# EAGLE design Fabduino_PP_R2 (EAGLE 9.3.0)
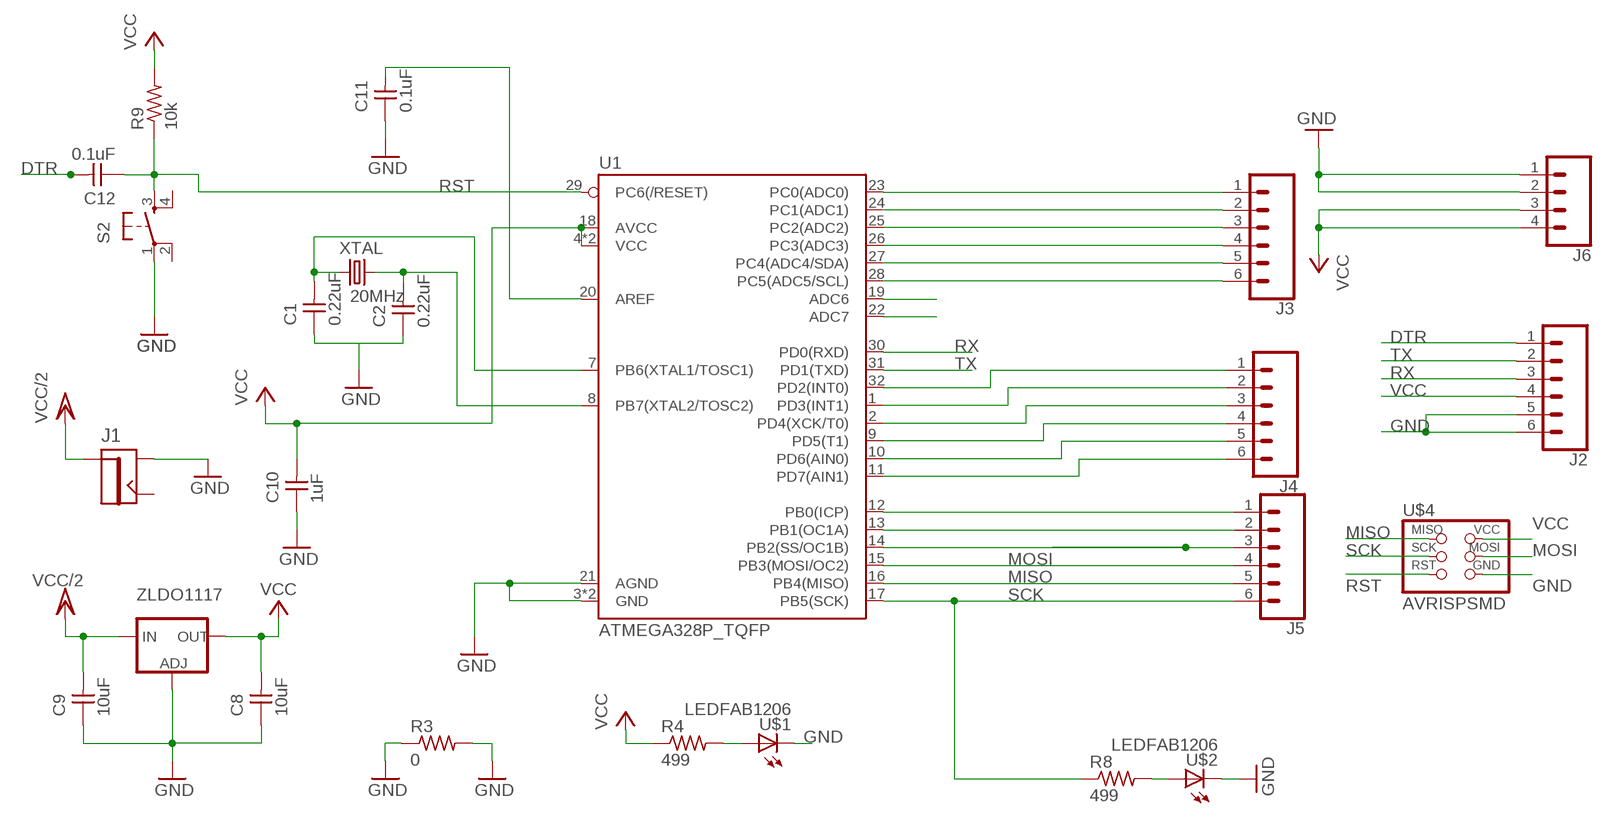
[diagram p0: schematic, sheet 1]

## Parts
C1  0.22uF  CAP-UNPOLARIZEDFAB  [C1206FAB]
C2  0.22uF  CAP-UNPOLARIZEDFAB  [C1206FAB]
C8  10uF  CAP-UNPOLARIZEDFAB  [C1206FAB]
C9  10uF  CAP-UNPOLARIZEDFAB  [C1206FAB]
C10  1uF  CAP-UNPOLARIZEDFAB  [C1206FAB]
C11  0.1uF  CAP-UNPOLARIZEDFAB  [C1206FAB]
C12  0.1uF  CAP-UNPOLARIZEDFAB  [C1206FAB]
J1  JACK.65MM  [JACK_.65MM]
J2  CONN_06SILK_FEMALE_PTH  [1X06]
J3  CONN_06SILK_FEMALE_PTH  [1X06]
J4  CONN_06SILK_FEMALE_PTH  [1X06]
J5  CONN_06SILK_FEMALE_PTH  [1X06]
J6  CONN_04PTH  [1X04]
R3  0  RES-US1206FAB  [R1206FAB]
R4  499  RES-US1206FAB  [R1206FAB]
R8  499  RES-US1206FAB  [R1206FAB]
R9  10k  RES-US1206FAB  [R1206FAB]
S2  6MM_SWITCH6MM_SWITCH  [6MM_SWITCH]
U1  ATMEGA328P_TQFP  [TQFP32-08]
U$1  LEDFAB1206  [LED1206FAB]
U$2  LEDFAB1206  [LED1206FAB]
U$4  AVRISPSMD  [2X03SMD]
XTAL  20MHz  CRYSTAL  [2-SMD-5X3MM]
ZLDO1117  V_REG_LM1117SOT223  [SOT223]

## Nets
DTR: C12.2 J2.1
GND: C1.1 C2.1 C8.1 C9.1 C10.1 C11.1 J1.CONTACT(SHUNT) J2.5 J2.6 J6.1 J6.2 R3.1 R3.2 S2.1(P) U1.3(GND) U1.5(GND) U1.21(AGND) U$1.2(C) U$2.2(C) U$4.6(GND) ZLDO1117.1(ADJ)
MISO: J5.5 U1.16(PB4(MISO)) U$4.1(MISO)
MOSI: J5.4 U1.15(PB3(MOSI/OC2)) U$4.4(MOSI)
N$2: J5.1 U1.12(PB0(ICP))
N$3: J3.1 U1.23(PC0(ADC0))
N$4: J3.2 U1.24(PC1(ADC1))
N$5: J3.3 U1.25(PC2(ADC2))
N$6: J3.4 U1.26(PC3(ADC3))
N$7: J3.5 U1.27(PC4(ADC4/SDA))
N$8: J3.6 U1.28(PC5(ADC5/SCL))
N$10: J4.1 U1.32(PD2(INT0))
N$11: J4.2 U1.1(PD3(INT1))
N$12: J4.3 U1.2(PD4(XCK/T0))
N$13: J4.4 U1.9(PD5(T1))
N$14: J4.5 U1.10(PD6(AIN0))
N$15: J4.6 U1.11(PD7(AIN1))
N$16: J5.2 U1.13(PB1(OC1A))
N$17: J5.3 U1.14(PB2(SS/OC1B))
N$18: C1.2 U1.7(PB6(XTAL1/TOSC1)) XTAL.P$1
N$19: C2.2 U1.8(PB7(XTAL2/TOSC2)) XTAL.P$2
N$20: C11.2 U1.20(AREF)
N$21: R4.2 U$1.1(A)
N$22: U1.19(ADC6)
N$23: R8.2 U$2.1(A)
N$24: U1.22(ADC7)
RST: C12.1 R9.1 S2.3(S) U1.29(PC6(/RESET)) U$4.5(RST)
RX: J2.3 U1.30(PD0(RXD))
SCK: J5.6 R8.1 U1.17(PB5(SCK)) U$4.3(SCK)
TX: J2.2 U1.31(PD1(TXD))
VCC: C8.2 C10.2 J2.4 J6.3 J6.4 R4.1 R9.2 U1.4(VCC) U1.6(VCC) U1.18(AVCC) U$4.2(VCC) ZLDO1117.2(OUT) ZLDO1117.4(OUT)
VCC/2: C9.2 J1.PIN ZLDO1117.3(IN)
Unconnected: J1.SHUNT(CONTACT) S2.2(P1) S2.4(S1)

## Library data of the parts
C1 C2 C8-C12 = fab:CAP-UNPOLARIZED
J1 = 01_fab:JACK
J2-J5 = SparkFun-Connectors:CONN_06: Multi connection point. Often used as Generic Header-pin footprint for 0.1 inch spaced/style header connections On any of the 0.1 inch spaced packages, you can populate with these: Break Away Headers - Straight (PRT-00116) Break Away Male Headers - Right Angle (PRT-00553) Female Headers (PRT-00115)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; PROD_ID: CONN-08437
J6 = SparkFun-Connectors:CONN_04: Multi connection point. Often used as Generic Header-pin footprint for 0.1 inch spaced/style header connections On any of the 0.1 inch spaced packages, you can populate with these: Break Away Headers - Straight (PRT-00116) Break Away Male Headers - Right Angle (PRT-00553) Female Headers (PRT-00115)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; PROD_ID: CONN-09696
R3 R4 R8 R9 = fab:RES-US: Resistor (US Symbol)
S2 = fab:6MM_SWITCH: OMRON SWITCH
U1 = SparkFun-IC-Microcontroller:ATMEGA328P_TQFP: Popular 328P in QFP Storefront component: ATmega328 - TQFP (COM-13448) Datasheet SparkFun Products SparkFun RedBoard - Programmed with Arduino (DEV-12757) Arduino Pro Mini 328 - 5V/16MHz (DEV-11113) Arduino Pro Mini 328 - 3.3V/8MHz (DEV-11114) SparkFun OpenLog (DEV-13712) SparkFun MicroView - OLED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; PROD_ID: IC-09069
U$1 U$2 = fab:LED: LED
U$4 = fab:AVRISP
XTAL = fab:CRYSTAL
ZLDO1117 = SparkFun-IC-Power:V_REG_LM1117: Voltage Regulator LM1117 Standard adjustable voltage regulator but in SMD form. Spark Fun Electronics SKU : COM-00595; PROD_ID: VREG-08170

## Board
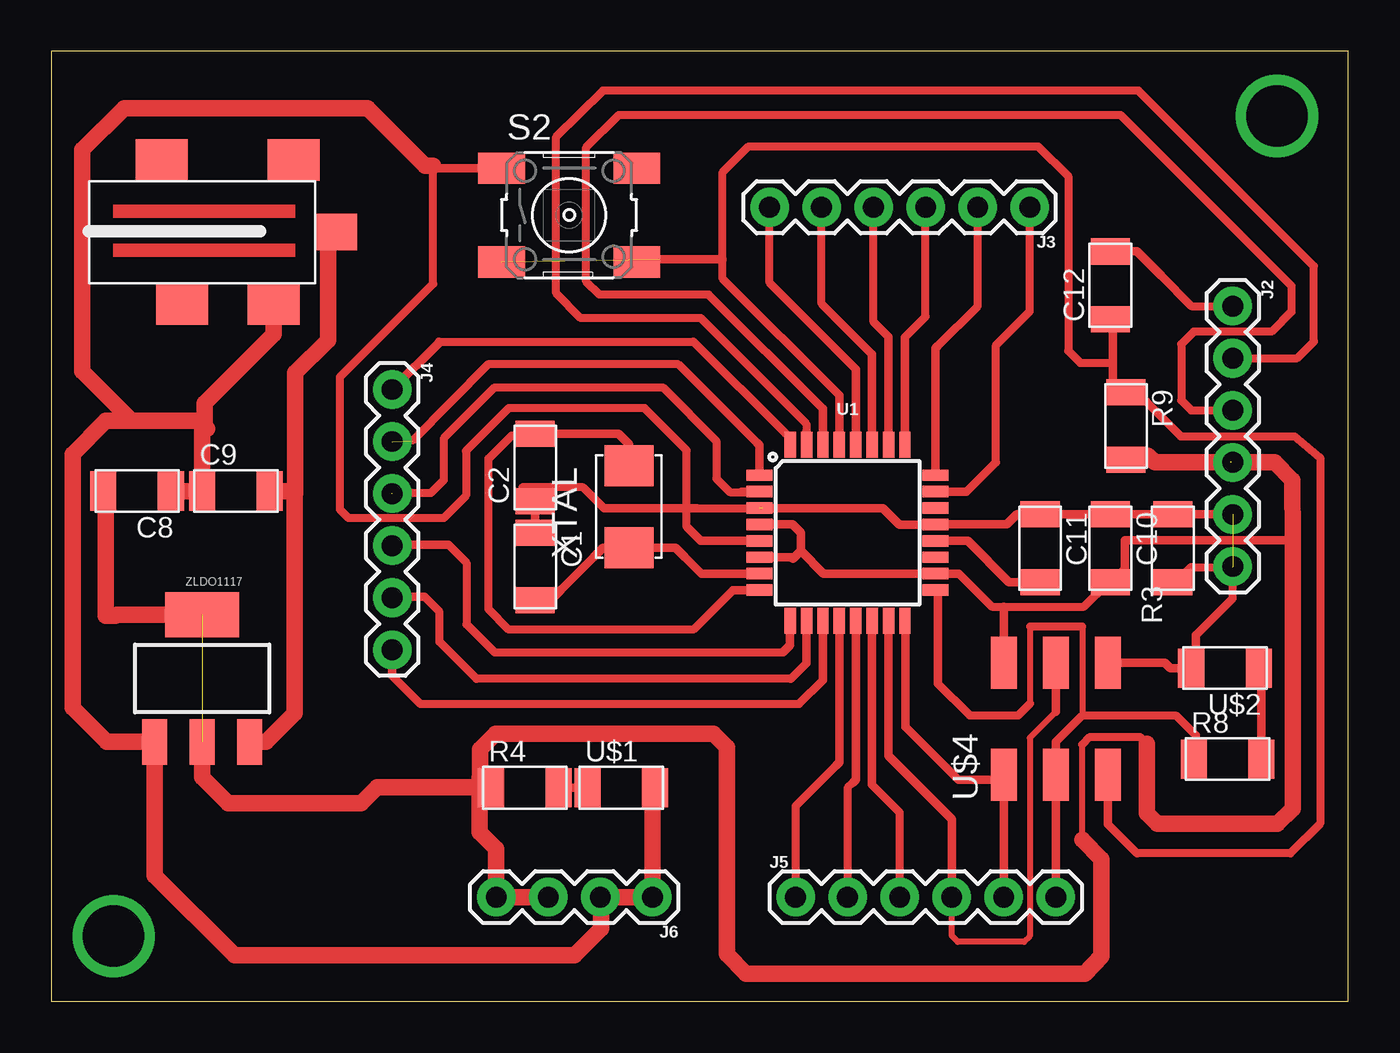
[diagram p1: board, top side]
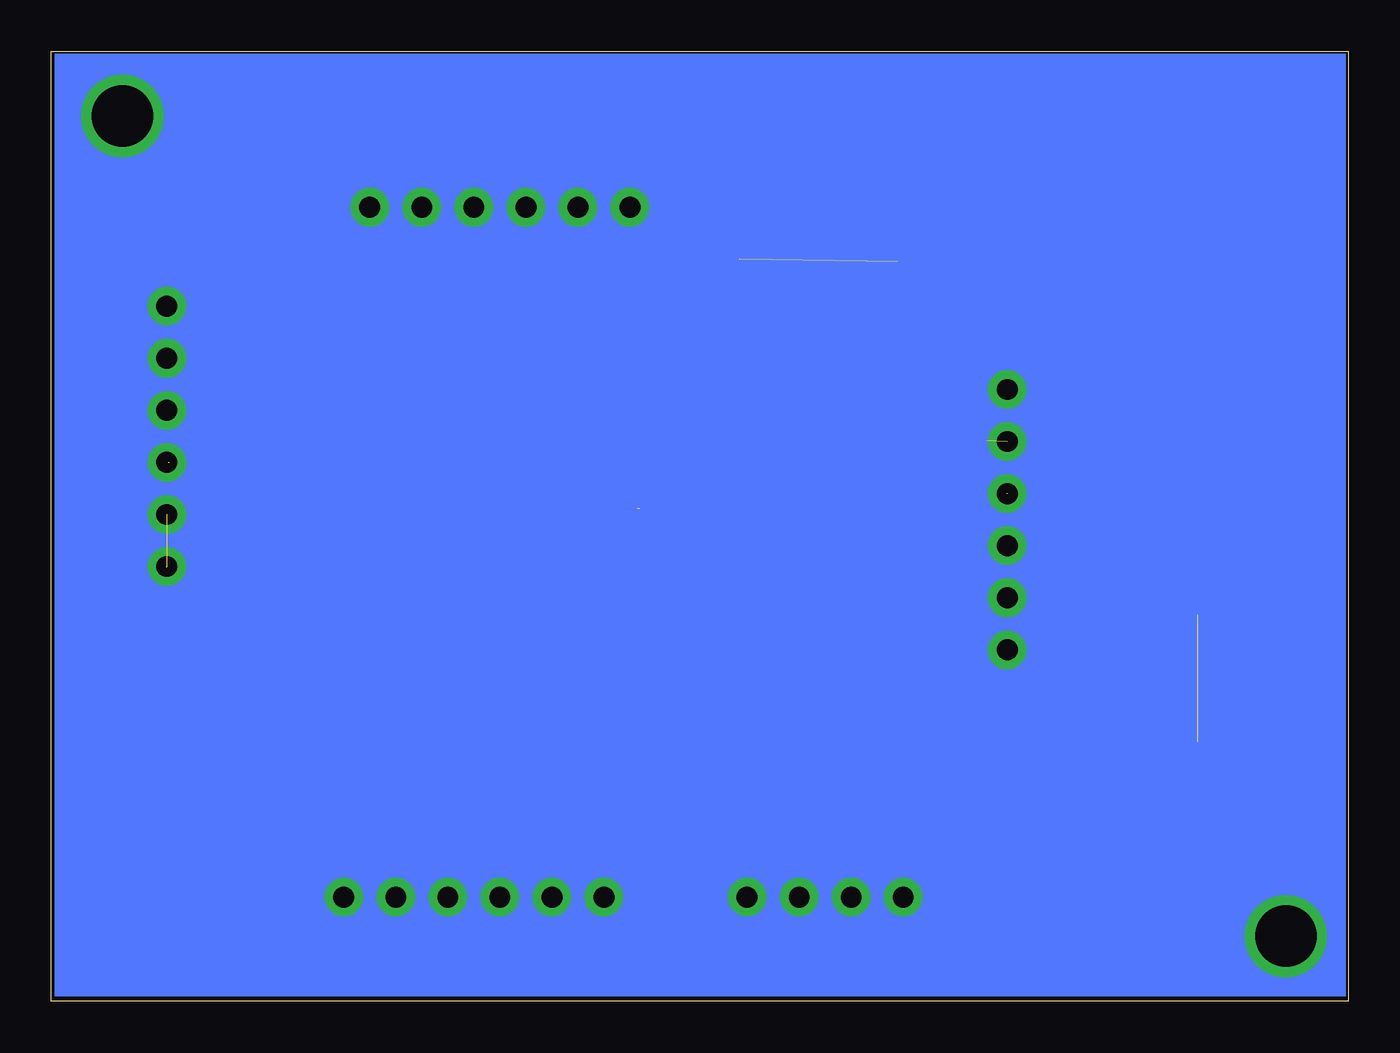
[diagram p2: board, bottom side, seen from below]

Size 63.3 x 46.34 mm. Coordinates in mm from the lower left corner, seen from the top.
Outline: 0,0 63.3,0 63.3,46.34 0,46.34 0,0
Copper layers (1*16): Top 0.035mm / dielectric 1.5mm / Bottom 0.035mm
Design rules "default": minimum track width 10mil, minimum drill 24mil, track to track 8mil, track to pad 8mil, pad to pad 8mil, via to via 8mil, smd to smd 8mil, copper to edge 40mil, drill to drill 8mil, minimum pad ring 10mil, minimum via ring 8mil, stop-mask expansion 4mil, vias tented up to drill 0mil, thermal gap 10mil

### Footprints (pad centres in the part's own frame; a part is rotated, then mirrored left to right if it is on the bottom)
C1206FAB = smd 1.27 x 1.905: 1 -1.651,0; 2 1.651,0
JACK_.65MM = smd 2.032 x 2.54: CONTACT 3.578,4.026; SHIELD -3.45,-1.448; SHIELD1 3.578,-0.447; SHUNT -3.45,5.005 | smd 1.778 x 2.032: PIN 0.064,7.071
1X06 = drill 1.016 pad 1.88: 1 0,0; 2 2.54,0; 3 5.08,0; 4 7.62,0; 5 10.16,0; 6 12.7,0
1X04 = drill 1.016 pad 1.88: 1 0,0; 2 2.54,0; 3 5.08,0; 4 7.62,0
R1206FAB = smd 1.27 x 1.905: 1 -1.651,0; 2 1.651,0
6MM_SWITCH = smd 2.286 x 1.524: 1 -3.302,2.286; 2 3.302,2.286; 3 -3.302,-2.286; 4 3.302,-2.286
TQFP32-08 = smd 1.27 x 0.559: 1 -4.293,2.8; 2 -4.293,2; 3 -4.293,1.2; 4 -4.293,0.4; 5 -4.293,-0.4; 6 -4.293,-1.2; 7 -4.293,-2; 8 -4.293,-2.8; 17 4.293,-2.8; 18 4.293,-2; 19 4.293,-1.2; 20 4.293,-0.4; 21 4.293,0.4; 22 4.293,1.2; 23 4.293,2; 24 4.293,2.8 | smd 0.559 x 1.27: 9 -2.8,-4.293; 10 -2,-4.293; 11 -1.2,-4.293; 12 -0.4,-4.293; 13 0.4,-4.293; 14 1.2,-4.293; 15 2,-4.293; 16 2.8,-4.293; 25 2.8,4.293; 26 2,4.293; 27 1.2,4.293; 28 0.4,4.293; 29 -0.4,4.293; 30 -1.2,4.293; 31 -2,4.293; 32 -2.8,4.293
LED1206FAB = smd 1.27 x 1.905: 1 -1.651,0; 2 1.651,0
2X03SMD = smd 2.54 x 1.27: 1 -2.54,2.54; 2 2.92,2.54; 3 -2.54,0; 4 2.92,0; 5 -2.54,-2.54; 6 2.92,-2.54
2-SMD-5X3MM = smd 2 x 2.4: P$1 -2,0; P$2 2,0
SOT223 = smd 1.219 x 2.235: 1 -2.311,-3.099; 2 0,-3.099; 3 2.311,-3.099 | smd 3.6 x 2.2: 4 0,3.099

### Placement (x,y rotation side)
C1  23.62,21.21 270 top
C2  23.62,26.04 90 top
C8  4.19,24.89 180 top
C9  9.02,24.89 0 top
C10  51.69,22.1 270 top
C11  48.26,22.1 270 top
C12  51.69,34.92 90 top
J1  6.83,37.59 270 top
J2  57.66,33.91 270 top
J3  47.75,38.73 180 top
J4  16.64,29.84 270 top
J5  36.32,5.08 0 top
J6  29.34,5.08 180 top
R3  54.74,22.1 90 top
R4  23.11,10.41 0 top
R8  57.4,11.81 0 top
R9  52.45,28.07 270 top
S2  25.27,38.35 0 top
U1  38.86,22.86 0 top
U$1  27.81,10.41 0 top
U$2  57.28,16.26 180 top
U$4  49.02,13.59 90 top
XTAL  28.19,24.13 90 top
ZLDO1117  7.37,15.75 0 top

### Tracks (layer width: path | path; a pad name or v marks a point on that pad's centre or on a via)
DTR
  Top 0.381: 54.17,35.38 55.63,33.91 J2.1
  Top 0.406: C12.2 52.98,36.58 54.17,35.38
GND  (3 unrouted)
  Top 0.254: U$1.2 29.46,9.02 29.34,8.89 | U$2.2 54.61,16.26 54.61,16.25
  Top 0.381: 26.82,5.08 J6.2 | 55.85,17.86 57.66,19.66 57.66,21.18 55.63,21.18 | 29.34,8.89 29.34,10.82 | 26.97,24.06 25.96,25.07 23.5,25.07 22.99,25.07 | 31.69,22.46 31.01,23.14 31.01,23.16 | 31.01,24.05 31.01,26.87 28.96,28.93 22.33,28.93 20.24,26.85 20.24,24.66 19.15,23.57 14.5,23.57 14.1,23.98 14.1,30.45 18.64,35 18.64,40.77 | 31.72,22.46 31.01,23.16 | 31.01,23.16 31.01,24.05 | 31.01,24.05 31.5,24.05 34.72,24.05
  Top 0.406: 55.85,16.25 54.61,16.25 54.36,16.51 U$4.6 | 51,23.75 51.56,23.75 | 51.56,23.75 53.09,23.75 | 53.09,23.75 54.1,23.75 | 54.1,23.75 55.24,23.75 | 55.24,23.75 J2.5 | 10.85,34.01 J1.CONTACT | C10.1 53.09,23.75 | 53.09,23.75 | 54.28,23.75 55.24,23.75 | R3.1 54.89,20.45 55.63,21.18 | R3.2 | R3.2 54.1,23.75 | C1.1 C2.1 23.5,24.51 23.5,25.07 | U$2.2 55.85,16.48 55.85,17.86 | 31.69,22.46 U1.5 | U1.3 40.58,24.06 41.4,23.24 43.14,23.24 U1.21 46.63,23.26 47.12,23.75 C11.1 51.56,23.75 | 51.56,23.75 | 26.97,24.06 31.49,24.06 31.5,24.05 | S2.1 18.36,40.64 18.24,40.77
  Top 0.813: 7.49,28.07 7.49,29.18 10.85,32.54 10.85,34.01 | 3.94,28.32 1.52,30.73 1.52,41.53 3.56,43.56 15.44,43.56 18.24,40.77 18.64,40.77 | 3.94,28.32 7.24,28.32 7.37,28.19 | 7.37,28.19 7.49,28.07 | 7.49,28.07 7.62,27.94 | 29.34,10.82 29.34,8.89 J6.1 26.82,5.08 26.82,3.53 25.53,2.23 8.94,2.23 5.05,6.12 ZLDO1117.1 2.72,12.65 1.04,14.33 1.04,26.7 2.67,28.32 3.94,28.32 | C8.1 C9.1 7.37,28.19
MISO
  Top 0.381: 41.68,13.39 44.27,10.79
  Top 0.406: 41.68,13.39 41.68,18.55 U1.16 | 44.27,10.79 46.23,10.79 U$4.1 J5.5
MOSI
  Top 0.305: 49.02,14.12 47.75,12.85 47.75,3.17 47.47,2.9 44.25,2.9 43.94,3.2 43.94,5.11
  Top 0.406: J5.4 43.94,5.11 43.94,8.89 40.86,11.97 U1.15 | U$4.4 49.02,14.12
N$1  (via drill 3 pad 2.18)
  other vias: 3.05,3.17
N$2
  Top 0.381: 38.49,11.69 38.29,11.49 36.32,9.53 J5.1
  Top 0.406: U1.12 38.46,11.66 38.29,11.49
N$3
  Top 0.381: 44.67,24.86 46.1,26.29 46.1,32 47.75,33.66 J3.1
  Top 0.406: U1.23 44.67,24.86
N$4
  Top 0.381: 43.28,31.98 45.21,33.91 J3.2
  Top 0.406: U1.24 43.16,31.85 43.28,31.98
N$5
  Top 0.381: 41.66,32.39 42.67,33.4 J3.3
  Top 0.406: 41.66,32.39 U1.25
N$6
  Top 0.381: 40.86,32.42 40.13,33.15 J3.4
  Top 0.406: U1.26 40.86,32.42
N$7
  Top 0.381: 40.06,31.57 37.59,34.04 J3.5
  Top 0.406: 40.06,31.57 U1.27
N$8
  Top 0.381: 39.26,30.84 35.05,35.05 J3.6
  Top 0.406: U1.28 39.26,30.84
N$9  (via drill 3 pad 2.18)
  other vias: 59.82,43.18
N$10
  Top 0.381: 18.92,32.18 31.34,32.18 35.83,27.7 36.09,27.43
  Top 0.406: U1.32 36.06,27.46 35.83,27.7 | J4.1 18.92,32.13 18.92,32.18
N$11  (1 unrouted)
  Top 0.381: 34.44,27.25 30.61,31.06 21.31,31.06 17.63,27.36
  Top 0.406: U1.1 34.57,27.13 34.44,27.25
N$12  (1 unrouted)
  Top 0.381: 34.7,24.84 33.66,24.84 33.12,24.84 32.46,25.5 32.46,27.33 29.84,29.95 21.64,29.95 19.15,27.46 19.15,25.43 18.52,24.79 16.64,24.79
  Top 0.406: U1.2 33.67,24.86 33.66,24.84
N$13
  Top 0.381: 19.38,22.28 20.27,21.39 20.27,18.39 21.64,17.02 35.71,17.02 36.07,17.37
  Top 0.406: U1.9 36.06,17.37 35.71,17.02 | J4.4 16.69,22.28 19.38,22.28
N$14
  Top 0.381: 36.86,16.49 36.09,15.72 20.75,15.72 18.95,17.53 18.95,19 18.21,19.74
  Top 0.406: U1.10 36.86,16.49 | J4.5 16.69,19.74 18.21,19.74
N$15
  Top 0.381: 37.67,15.67 36.5,14.5 18.01,14.5 16.64,15.88
  Top 0.406: U1.11 37.66,15.68 37.67,15.67 | 16.64,15.88 J4.6
N$16
  Top 0.381: 39.12,10.67 38.86,10.41 J5.2
  Top 0.406: U1.13 39.26,10.81 39.12,10.67
N$17
  Top 0.381: 40.06,10.56 41.4,9.22 J5.3
  Top 0.406: U1.14 40.06,10.56
N$18
  Top 0.381: 26.47,21.67 24.88,20.08 24.61,19.81 | 30.94,21.67 31.74,20.86
  Top 0.406: C1.2 24.36,19.56 24.88,20.08 | U1.7 31.74,20.86 | 26.47,21.67 26.93,22.13 XTAL.P$1 30.47,22.13 30.94,21.67
N$19
  Top 0.381: 33.27,20.06 31.34,18.14 22.33,18.14 21.34,19.13 21.34,26.47 22.45,27.58
  Top 0.406: 22.45,27.58 23.52,27.58 C2.2 27.69,27.69 28.19,27.18 XTAL.P$2 | U1.8 33.27,20.06
N$20
  Top 0.406: U1.20 44.72,22.46 46.74,20.45 C11.2
N$21
  Top 0.406: 26.47,10.41 U$1.1 R4.2
N$23
  Top 0.406: R8.2 59.05,14.86 59.05,15.9 59.05,16.13 U$2.1
RST  (1 unrouted)
  Top 0.381: 38.46,29.56 32.77,35.26 32.77,36.2 32.77,40.44 34.04,41.71 48.16,41.71 49.63,40.26 49.63,31.73 50.22,31.14 51.82,31.14 51.82,30.1 | 51.82,29.44 51.79,29.41 | 52.98,29.69 53.47,29.21 55.12,27.56 60.68,27.56 61.92,26.52 61.92,8.66 60.48,7.21 52.98,7.21 51.56,8.64
  Top 0.406: C12.1 51.82,33.15 51.82,30.1 | 51.82,30.1 51.82,29.44 | 53.47,29.21 52.96,29.72 R9.1 52.2,29.72 51.82,30.1 | U1.29 38.46,29.56 | 29.72,36.2 32.77,36.2 | 51.56,8.64 U$4.5
RX
  Top 0.381: J2.3 55.63,28.83 55.14,29.31 55.14,32.05 55.75,32.66 59.56,32.66 60.53,33.63 60.53,34.9 52.2,43.23 27.69,43.23 26.11,41.66 26.11,35.1 26.75,34.47 32.08,34.47 37.66,28.91
  Top 0.406: U1.30 37.66,28.91
SCK
  Top 0.305: 47.78,14.53 47.78,18.29 | 50.32,18.29 50.32,13.92
  Top 0.381: 55.85,12.98 54.91,13.92 50.32,13.92 50.27,13.89 49.02,12.65 | 43.28,15.49 44.83,13.95 47.19,13.95 47.78,14.53 | 47.78,18.29 50.32,18.29
  Top 0.406: R8.1 55.85,11.91 55.85,12.98 | 43.28,15.49 43.28,19.93 U1.17 | 49.02,12.65 U$4.3 J5.6
TX
  Top 0.381: J2.2 60.81,31.37 61.62,32.18 61.62,35.87 53.06,44.42 26.92,44.42 24.64,42.16 24.64,34.54 25.83,33.33 31.7,33.33 36.85,28.17 36.85,27.81 36.85,27.03
  Top 0.406: U1.31 36.85,27.81
VCC  (2 unrouted)
  Top 0.305: 50.32,7.87 50.32,12.52
  Top 0.381: 57.53,26.29 J2.4 | 20.9,10.92 20.93,10.44 | 44.29,20.86 45.9,19.25 46.48,19.25 50.39,19.25 51,19.86 | 50.32,12.52 50.7,12.9 53.14,12.9 53.47,12.57 | 60.38,22.48 60.58,22.48
  Top 0.406: 52.4,20.8 52.4,21.08 | 52.4,21.08 52.4,22.48 60.38,22.48 | 51,19.86 51.59,20.45 C10.2 51.77,20.45 52.4,21.08 | R9.2 53.72,26.42 53.85,26.29 | R4.1 20.95,10.41 20.93,10.44 | U1.4 36.18,23.26 36.58,22.86 36.58,21.97 | 36.58,21.97 36.2,21.59 36.12,21.66 U1.6 | 36.58,21.97 37.69,20.86 U1.18 44.29,20.86 | U$4.2 46.48,19.25
  Top 0.813: 57.53,26.29 53.85,26.29 53.52,26.62 51.87,26.62 | J6.3 J6.4 21.72,7.44 20.9,8.26 20.9,10.92 | 50.32,7.87 51.26,6.93 51.26,2.18 50.44,1.35 33.91,1.35 32.97,2.29 32.97,12.39 32.31,13.06 21.69,13.06 20.93,12.29 20.93,10.44 15.9,10.44 15.11,9.65 8.64,9.65 7.37,10.92 ZLDO1117.2 | 53.47,12.57 53.47,9.17 53.98,8.66 59.84,8.66 60.58,9.4 60.58,22.48 60.55,25.43 59.72,26.29 57.58,26.29 | ZLDO1117.4 3.2,18.85 3.15,18.8 2.67,18.8 2.67,24.77 C8.2
VCC/2
  Top 0.406: 13.51,37.36 13.58,37.53 J1.PIN
  Top 0.813: 11.91,24.77 11.89,24.74 11.89,14.05 10.49,12.65 ZLDO1117.3 | 11.91,24.77 11.91,30.66 13.51,32.26 13.51,37.36 | C9.2 11.79,24.89 11.91,24.77
(copper drawn outside any net)
  shapes: Bottom area x1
